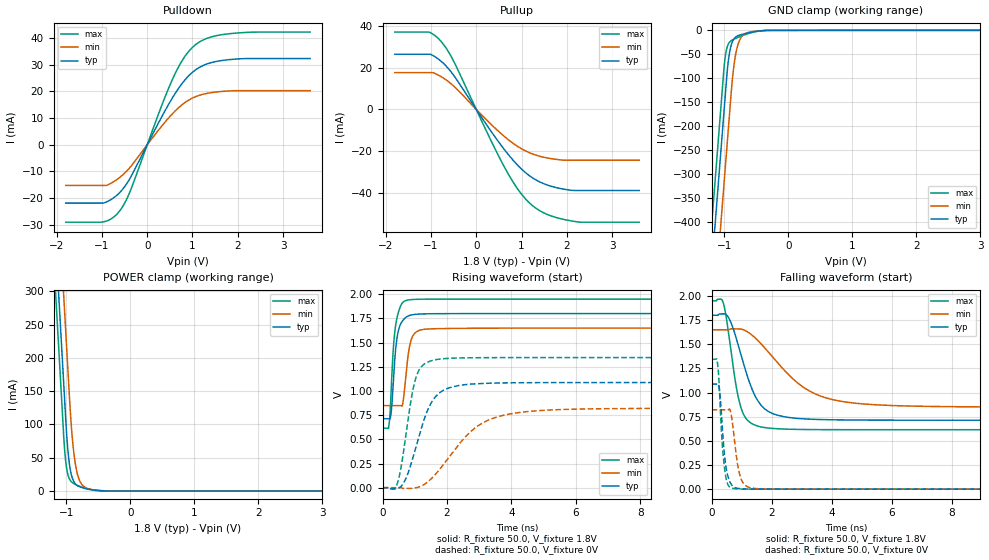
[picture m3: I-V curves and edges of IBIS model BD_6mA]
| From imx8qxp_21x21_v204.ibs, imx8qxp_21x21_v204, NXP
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[Model]   BD_6mA
Model_type I/O
Polarity   Non-Inverting
Enable   Active-Low
| C_comp min and max val. don't necessarily correlate with the min and max pvt
| but are the smallest and greatest pad capacitance found.
| var   typ   min   max
C_comp   1.59280pF  1.51795pF  1.66135pF
Vinl = 577.5mV
Vinh = 1.2675V
Vmeas = 900.0mV   | Reference voltage for timing measurements
Cref  = 15.0pF   | Timing specification test load capacitance value
Rref  = 1.0MOhm   | Timing specification test load resistance value
Vref  = 1.8V   | Timing specification test load voltage
[Model Spec]
| :
Vinl 630.00000mV 577.50000mV 682.50000mV
Vinh 1.17000V 1.07250V 1.26750V
| variable   typ   min   max
[Temperature Range] 25.0 125.0 -40.0
| variable   typ   min   max
[Voltage Range] 1.8V 1.65V 1.95V
| variable   typ   min   max
[POWER Clamp Reference] 1.8V 1.65V 1.95V
| variable   typ   min   max
[GND Clamp Reference] 0V 0V 0V
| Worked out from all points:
|   slope of the pulldown table from 0 to 0.27 V, typ, clamps not added: 30.5 ohm
|   slope of the pullup table from 0 to 0.27 V, typ, clamps not added: 31.2 ohm
|   GND clamp passes 1 mA (typ) near -0.44 V on its own axis
|   POWER clamp passes 1 mA (typ) near -0.55 V on its own axis
|   rising waveform, R_fixture 50.0, V_fixture 1.8V: 20-80 % time 161ps typ, 177ps min, 157ps max; typ from 0.714 V to 1.8 V
|   falling waveform, R_fixture 50.0, V_fixture 1.8V: 20-80 % time 708ps typ, 1.61ns min, 408ps max; typ from 1.8 V to 0.714 V
|   rising waveform, R_fixture 50.0, V_fixture 0V: 20-80 % time 640ps typ, 1.33ns min, 382ps max; typ from 0 V to 1.09 V
|   falling waveform, R_fixture 50.0, V_fixture 0V: 20-80 % time 176ps typ, 217ps min, 158ps max; typ from 1.09 V to 0 V
[POWER Clamp]
-1.8V     1.452A     1.584A     1.373A
-1.18V    398.2mA    529.9mA    318.8mA
-1.15V    347.2mA    478.9mA    267.8mA
-1.12V    296.2mA    427.9mA    216.8mA
-1.04V    160.2mA    291.9mA    80.78mA
-1V       92.69mA    223.9mA    36.89mA
-950mV    39.12mA    138.9mA    17.72mA
-890mV    15.28mA    63.28mA    11.47mA
-820mV    7.619mA    23.03mA    8.072mA
-710mV    3.877mA    5.679mA    4.137mA
-440mV    198.6uA    468.9uA    81.6uA
3.6V      0A         0A         0A
[GND Clamp]
-1.8V     -1.52A     -1.672A    -1.429A
-1.21V    -517.1mA   -668.6mA   -425.9mA
-1.12V    -364.1mA   -515.6mA   -272.9mA
-1.04V    -228.1mA   -379.6mA   -136.9mA
-990mV    -143.1mA   -294.6mA   -59.11mA
-960mV    -92.41mA   -243.6mA   -36.73mA
-930mV    -55.69mA   -192.6mA   -26.66mA
-870mV    -22.37mA   -96.04mA   -19.77mA
-810mV    -12.81mA   -41.2mA    -16.04mA
-700mV    -7.565mA   -8.808mA   -10.1mA
-450mV    -1.118mA   -1.064mA   -1.253mA
3.6V      32.66uA    16.11uA    55.52uA
| variable   typ   min   max
[Pullup Reference] 1.8V 1.65V 1.95V
| variable   typ   min   max
[Pulldown Reference] 0V 0V 0V
[Pullup]
-1.8V     26.35mA    17.57mA    36.94mA
-1.04V    26.35mA    17.57mA    36.94mA
-950mV    25.67mA    17.57mA    35.85mA
-740mV    22.3mA     15.17mA    31.51mA
-450mV    14.82mA    10.19mA    20.91mA
310mV     -9.916mA   -6.764mA   -14.18mA
650mV     -19.99mA   -13.44mA   -28.64mA
990mV     -28.3mA    -18.69mA   -40.24mA
1.24V     -32.67mA   -21.27mA   -45.94mA
1.65V     -36.69mA   -23.52mA   -50.87mA
2.17V     -38.75mA   -24.29mA   -53.53mA
3.6V      -38.75mA   -24.29mA   -53.9mA
[Pulldown]
-1.8V     -21.86mA   -15.25mA   -29.02mA
-960mV    -21.81mA   -15.25mA   -28.88mA
-790mV    -20.44mA   -14.32mA   -27.72mA
-600mV    -17.76mA   -12.13mA   -24.6mA
-370mV    -12.26mA   -8.28mA    -17.15mA
310mV     10.15mA    6.783mA    14.27mA
570mV     17.95mA    11.86mA    25mA
820mV     24.05mA    15.66mA    32.85mA
1.07V     28.12mA    18.05mA    37.56mA
1.33V     30.36mA    19.3mA     39.96mA
1.8V      31.9mA     20.17mA    41.6mA
3.6V      32.32mA    20.28mA    42.24mA
[Ramp]
dV/dt_r 652.1386mV/639.7079ps 492.69392mV/1.3349ns 807.00499mV/381.55933ps
dV/dt_f 651.73726mV/708.24755ps 480.29898mV/1.60745ns 800.78636mV/407.83562ps
R_load = 50.0
| Removed startup time: 0s 0s 0s  .
| Removed end time: 20.0ns.
[Rising Waveform]
R_fixture   = 50.0
V_fixture   = 1.8V
V_fixture_min = 1.65V
V_fixture_max = 1.95V
0s        714mV      849.6mV    615.5mV
192ps     714.2mV    849.6mV    628.2mV
276ps     804mV      849.6mV    1.065V
376ps     1.309V     849.6mV    1.598V
468ps     1.585V     849.6mV    1.784V
608ps     1.719V     847.2mV    1.907V
792ps     1.775V     1.363V     1.94V
996ps     1.791V     1.596V     1.947V
1.492ns   1.798V     1.642V     1.949V
20ns      1.8V       1.65V      1.95V
| Removed startup time: 0s 0s 0s  .
| Removed end time: 20.0ns.
[Falling Waveform]
R_fixture   = 50.0
V_fixture   = 1.8V
V_fixture_min = 1.65V
V_fixture_max = 1.95V
0s        1.8V       1.65V      1.95V
400ps     1.814V     1.65V      1.917V
596ps     1.758V     1.652V     1.547V
820ps     1.564V     1.66V      1.064V
1.028ns   1.339V     1.653V     800.8mV
1.36ns    1.026V     1.591V     675.1mV
1.664ns   864mV      1.499V     642.9mV
3.1ns     727.5mV    1.046V     617.4mV
4.656ns   715.7mV    893.8mV    615.2mV
20ns      713.8mV    849.5mV    615.4mV
| Removed startup time: 0s 0s 0s  .
| Removed end time: 20.0ns.
[Rising Waveform]
R_fixture   = 50.0
V_fixture   = 0V
V_fixture_min = 0V
V_fixture_max = 0V
0s        299.2nV    664.2nV    758.6nV
440ps     -10.23mV   617nV      28.31mV
564ps     10.75mV    1.005mV    191.2mV
720ps     92.27mV    -8.061mV   532.9mV
1.028ns   410.2mV    -968.9uV   1.128V
1.356ns   765.7mV    48.51mV    1.29V
1.628ns   934.5mV    133.1mV    1.322V
2.936ns   1.075V     633.4mV    1.344V
4.384ns   1.086V     783.2mV    1.345V
20ns      1.087V     821.2mV    1.345V
| Removed startup time: 0s 0s 0s  .
| Removed end time: 20.0ns.
[Falling Waveform]
R_fixture   = 50.0
V_fixture   = 0V
V_fixture_min = 0V
V_fixture_max = 0V
0s        1.087V     821mV      1.345V
208ps     1.091V     821mV      1.279V
280ps     980.2mV    821mV      905.8mV
356ps     652.2mV    821mV      462.8mV
468ps     253.7mV    821mV      137.6mV
612ps     74.99mV    825.1mV    20.48mV
720ps     27.38mV    627mV      7.416mV
980ps     4.42mV     109.1mV    1.312mV
1.448ns   743.6uV    7.215mV    349.8uV
20ns      354.7nV    750.5nV    800nV
